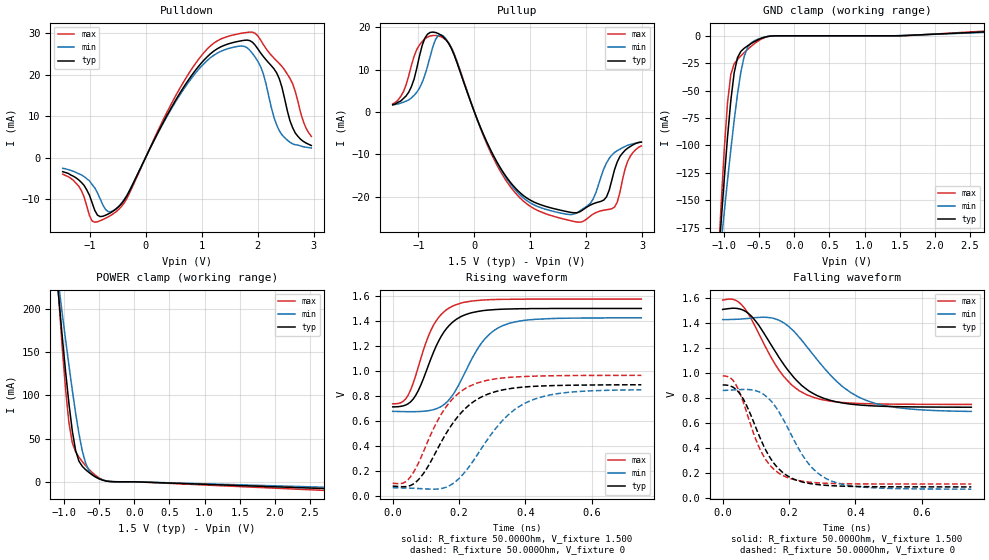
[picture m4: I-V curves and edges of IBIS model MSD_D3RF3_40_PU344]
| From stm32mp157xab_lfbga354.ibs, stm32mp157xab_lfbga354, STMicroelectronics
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[Model] MSD_D3RF3_40_PU344
Model_type   I/O
C_comp 2.329pF   2.247pF   2.450pF
Vinh = 925.000mV
Vinl = 575.000mV
Vmeas = 750.000mV
Vref = 750.000mV
[Model Spec]
Vinh   925.000mV   888.000mV   963.000mV
Vinl   575.000mV   538.000mV   613.000mV
Vmeas   750.000mV   713.000mV   788.000mV
Vref   750.000mV   713.000mV   788.000mV
[Temperature Range]   25.000   125.000   -40.000
[Voltage Range]   1.500V   1.425V   1.575V
[GND Clamp Reference]   0.00V   0.00V   0.00V
[Pulldown Reference]   0.00V   0.00V   0.00V
[POWER Clamp Reference]   1.500V   1.425V   1.575V
[Pullup Reference]   1.500V   1.425V   1.575V
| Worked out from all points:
|   slope of the pulldown table from 0 to 0.225 V, typ, clamps not added: 36.6 ohm
|   slope of the pullup table from 0 to 0.225 V, typ, clamps not added: 31.2 ohm
|   GND clamp passes 1 mA (typ) near -0.40 V on its own axis
|   POWER clamp passes 1 mA (typ) near -0.41 V on its own axis
|   rising waveform, R_fixture 50.000Ohm, V_fixture 1.500: 20-80 % time 81.4ps typ, 98.8ps min, 70.7ps max; typ from 0.714 V to 1.5 V
|   rising waveform, R_fixture 50.000Ohm, V_fixture 0: 20-80 % time 123ps typ, 141ps min, 107ps max; typ from 0.081 V to 0.891 V
|   falling waveform, R_fixture 50.000Ohm, V_fixture 1.500: 20-80 % time 130ps typ, 156ps min, 114ps max; typ from 1.5 V to 0.723 V
|   falling waveform, R_fixture 50.000Ohm, V_fixture 0: 20-80 % time 90.7ps typ, 108ps min, 79ps max; typ from 0.901 V to 0.086 V
[GND Clamp]
-1.48V    -593.8mA   -479.5mA   -763mA
-1.098V   -218.2mA   -223.3mA   -220.2mA
-1.05V    -174mA     -192.3mA   -159.6mA
-1.002V   -131.9mA   -161.9mA   -105.2mA
-954.6mV  -92.79mA   -132.2mA   -61.49mA
-906.8mV  -58.98mA   -103.9mA   -35.12mA
-859.1mV  -33.77mA   -77.12mA   -25.6mA
-811.4mV  -19.87mA   -53.03mA   -21.59mA
-715.9mV  -11.38mA   -18.7mA    -15.38mA
-572.7mV  -5.4mA     -4.611mA   -7.303mA
-286.4mV  -62.82uA   -108.6uA   -50.82uA
2.959V    4.272mA    3.643mA    5.154mA
[Power Clamp]
-1.459V   577.6mA    479.2mA    722.9mA
-1.077V   211mA      225.5mA    210.3mA
-1.03V    168.2mA    194.7mA    155.6mA
-981.8mV  127.5mA    164.3mA    106.7mA
-934.1mV  90.5mA     134.7mA    68.26mA
-886.4mV  59.02mA    106.2mA    45.17mA
-838.6mV  36.17mA    79.41mA    34.61mA
-743.2mV  17.86mA    35.55mA    23.3mA
-647.7mV  10.74mA    12.84mA    14.33mA
-552.3mV  5.478mA    5.433mA    7.218mA
-313.6mV  101.8uA    235.2uA    114.2uA
2.98V     -8.607mA   -6.939mA   -10.98mA
[Pulldown]
-1.48V    -3.4mA     -2.6mA     -4mA
-1.193V   -5.4mA     -3.9mA     -6.9mA
-954.6mV  -10.91mA   -6.5mA     -15.28mA
-811.4mV  -14.22mA   -9.94mA    -15.22mA
-525mV    -12.36mA   -12.3mA    -13.02mA
906.8mV   21.31mA    20.61mA    22.95mA
1.289V    26.28mA    25.21mA    28.18mA
1.766V    28.25mA    26.78mA    30.06mA
2.052V    25.24mA    21.95mA    28.34mA
2.434V    16.97mA    5.5mA      21.96mA
2.673V    5.9mA      3.1mA      15.9mA
2.959V    2.9mA      2.3mA      5.1mA
[Pullup]
-1.459V   1.7mA      1.714mA    1.929mA
-1.173V   4.7mA      2.871mA    8.571mA
-981.8mV  13.2mA     5.629mA    15.84mA
-838.6mV  18.38mA    10.73mA    17.71mA
-552.3mV  17.7mA     17.93mA    17.47mA
640.9mV   -16.58mA   -16.97mA   -17.61mA
1.834V    -23.79mA   -23.78mA   -25.99mA
2.12V     -21.68mA   -20.55mA   -24.11mA
2.311V    -20.78mA   -13.38mA   -23.19mA
2.502V    -13.6mA    -9.557mA   -22.45mA
2.741V    -8.5mA     -7.829mA   -11.5mA
2.98V     -7.1mA     -7.1mA     -8.014mA
[Ramp]
R_load=50.000Ohm
dV/dt_r   474.957mV/102.500ps  457.947mV/121.500ps  506.160mV/89.000ps
dV/dt_f   474.957mV/110.500ps  457.947mV/134.000ps  506.160mV/97.500ps
[Rising waveform]
R_fixture=50.000Ohm
V_fixture=1.500
V_fixture_min=1.425
V_fixture_max=1.575
0s        714mV      678.1mV    738.2mV
39ps      728.4mV    675.8mV    777.2mV
62ps      777.3mV    675.6mV    904.8mV
123ps     1.151V     691.8mV    1.367V
154ps     1.311V     731.3mV    1.472V
184ps     1.398V     821.1mV    1.523V
268ps     1.481V     1.225V     1.567V
330ps     1.494V     1.361V     1.573V
429ps     1.499V     1.413V     1.575V
749ps     1.5V       1.425V     1.575V
[Rising waveform]
R_fixture=50.000Ohm
V_fixture=0
0s        81.13mV    67.48mV    104.1mV
39ps      76.76mV    65.69mV    115.7mV
77ps      131.1mV    61.75mV    262.1mV
154ps     470.2mV    66.13mV    687.8mV
192ps     622.2mV    123.2mV    807.7mV
230ps     727.8mV    235.5mV    877.3mV
330ps     848.8mV    603mV      944.4mV
406ps     874.6mV    752.7mV    957.3mV
521ps     886mV      827.7mV    963.7mV
749ps     890.5mV    850.1mV    965.5mV
[Falling waveform]
R_fixture=50.000Ohm
V_fixture=1.500
V_fixture_min=1.425
V_fixture_max=1.575
0s        1.505V     1.424V     1.58V
46ps      1.512V     1.427V     1.568V
85ps      1.455V     1.436V     1.434V
177ps     1.092V     1.408V     992.4mV
207ps     985.1mV    1.349V     902.6mV
253ps     866.2mV    1.209V     822.7mV
345ps     764.5mV    925.5mV    764.7mV
429ps     737.4mV    781.2mV    751.4mV
552ps     726.4mV    711.9mV    746.8mV
749ps     723.1mV    689.4mV    745.1mV
[Falling waveform]
R_fixture=50.000Ohm
V_fixture=0
0s        901.1mV    856.6mV    973mV
23ps      892.6mV    859.9mV    957.8mV
46ps      849.8mV    863.4mV    871.4mV
115ps     463mV      839.1mV    372.6mV
154ps     275.5mV    745.9mV    227.2mV
192ps     179mV      578mV      163.8mV
253ps     117.3mV    290.1mV    126.4mV
330ps     95.21mV    130.1mV    113.2mV
452ps     87.31mV    78.87mV    109.3mV
749ps     85.77mV    67.64mV    108.7mV
